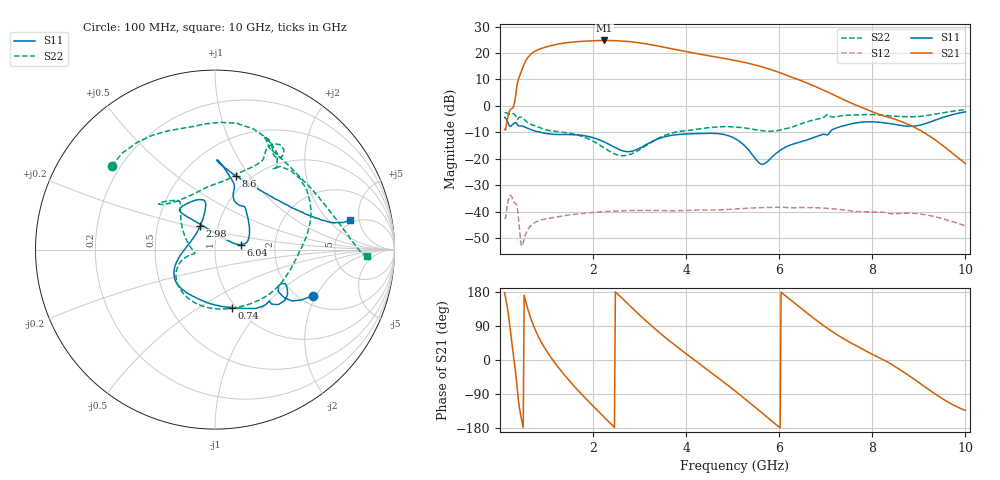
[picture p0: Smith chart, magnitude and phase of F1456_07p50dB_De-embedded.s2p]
! Integrated Device Technology
! Corporate Headquarters
! 6024 Silver Creek Valley Road
! San Jose, CA 95138  USA
! Phone:  1-408-284-8200
! Toll Free:  1-800-223-1366
! Webpage:  http://www.idt.com/
! Timing and RF Division
! 515 Groton Road, Suite 102
! Westford, MA 01886-6024
! Device:  F1456
! Description: 6-bit 0.5 dB Transmit Variable Gain Amplifier
! Frequency:  2100.0 -  2950.00 MHz
! Package:  6x6 mm Thin QFN Plastic Package: 28 pin
! State:  15
! Atten State:  7.5 dB
! Voltage:  +5.00 Volts
! Current:  217.036 mA
! Data:  The device was measured on a the F1455 evaluation board which has
!  individual transmission lines to the RF pins.  Data was collected
!  using a calibrated network analyzer.  The evaluation board was
!  de-embedded using a TRL calibration technique.
!  The reference plane is the edge of the package pin.
!  Pin  1 = CSb
!  Pin  2 = DATA
!  Pin  3 = CLK
!  Pin  4 = RSET
!  Pin  5 = GND
!  Pin  6 = RFIN  = Port 1
!  Pin  7 = GND
!  Pin  8 = NC
!  Pin  9 = NC
!  Pin 10 = NC
!  Pin 11 = NC
!  Pin 12 = NC
!  Pin 13 = NC
!  Pin 14 = /STBY
!  Pin 15 = GND
!  Pin 16 = RFOUT  = Port 2
!  Pin 17 = GND
!  Pin 18 = NC
!  Pin 19 = NC
!  Pin 20 = NC
!  Pin 21 = GND
!  Pin 22 = NC
!  Pin 23 = GND
!  Pin 24 = NC
!  Pin 25 = NC
!  Pin 26 = NC
!  Pin 27 = GND
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# GHz S dB R 50
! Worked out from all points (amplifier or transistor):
!   496 points, 100 MHz to 10 GHz, reference 50 ohm
!   highest |S21| = 24.7 dB at 2.24 GHz (marker M1)
!   |S21| within 3 dB of that: 894.4 MHz to 3.648 GHz (2.754 GHz wide, 121 % of centre)
!   unconditionally stable (mu >= 1): start of sweep to end of sweep
!   at 1.74 GHz: K = 2.94, MAG = 25.0 dB, |S12| = -40.7 dB
!   at 5.06 GHz: K = 5.02, MAG = 18.1 dB, |S12| = -39.0 dB
!   at 10 GHz: K = 133.74, MAG = -12.5 dB, |S12| = -45.4 dB
!   S11 on the Smith chart (normalised r, x): 100 MHz: 2.34, -1.91; 740 MHz: 0.96, -0.70; 2.98 GHz: 0.82, +0.22; 6.04 GHz: 1.34, +0.08; 8.6 GHz: 0.86, +0.87; 10 GHz: 4.61, +3.73
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0.1  -4.35 -25.2  -8.90 177.8  -42.39 44.7  -2.61 141.0
0.32  -6.44 -32.0  1.88 -16.5  -36.77 -133.9  -3.32 64.0
0.42  -7.60 -43.3  11.19 -127.6  -46.58 140.2  -4.28 46.1
0.56  -8.20 -57.6  17.21 151.7  -48.22 -176.1  -5.76 8.2
0.74  -9.44 -73.4  20.54 84.8  -44.23 136.8  -7.50 -21.5
0.98  -10.39 -95.3  22.21 28.2  -42.75 91.0  -9.01 -60.7
1.2  -10.82 -113.0  23.18 -10.7  -42.08 65.5  -9.66 -91.0
1.5  -10.85 -131.6  24.00 -56.0  -41.22 39.2  -10.36 -124.6
1.76  -11.15 -144.3  24.40 -91.0  -40.70 20.9  -11.52 -145.0
2.24  -13.65 -167.1  24.73 -151.0  -40.02 -8.1  -15.90 -166.2
2.58  -16.65 166.6  24.57 167.9  -39.73 -27.0  -18.78 -169.1
2.98  -16.18 122.0  23.86 121.0  -39.55 -47.9  -16.76 170.0
3.4  -12.49 102.9  22.61 74.9  -39.59 -68.4  -12.29 140.4
3.74  -11.01 102.7  21.40 40.7  -39.68 -83.1  -10.07 128.2
4.1  -10.57 112.8  20.16 7.2  -39.51 -97.7  -9.17 128.5
4.6  -10.39 129.8  18.63 -39.1  -39.37 -119.2  -8.06 137.9
5.06  -12.45 130.1  17.14 -82.6  -39.00 -138.7  -7.99 140.7
6.04  -16.58 10.8  12.37 178.6  -38.28 168.1  -9.06 96.2
6.7  -12.27 39.9  7.88 113.9  -38.47 129.6  -5.53 63.8
8.36  -6.63 84.4  -4.36 -7.3  -40.71 55.7  -3.79 62.4
8.6  -7.36 74.2  -5.78 -26.1  -40.67 49.5  -4.02 55.7
10  -2.27 12.3  -21.86 -132.5  -45.36 -29.5  -1.46 -2.5
